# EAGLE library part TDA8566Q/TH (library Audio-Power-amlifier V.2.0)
The TDA8566Q is an integrated class-B output amplifier contained in a 17-lead single-in-line (SIL; bent to DIL) plastic power package. The device contains two amplifiers in a Bridge-Tied Load configuration (BTL). The output power is 2 ´ 25 W in a 4 W load or 2 ´ 40 W in a 2 W load. It has a differential input stage and two diagnostic outputs. The device is primarily developed for car radio applications. The TDA8566TH is an integrated class-B output amplifier contained in a 20-lead small outline plastic package. The device contains 2 amplifiers in a Bridge-Tied Load (BTL) configuration. The output power is 2 ´ 25 W in a 4 W load or 2 ´ 40 W in a 2 W load. It has a differential input stage and 2 diagnostic outputs. The device is primarily developed for car radio applications.
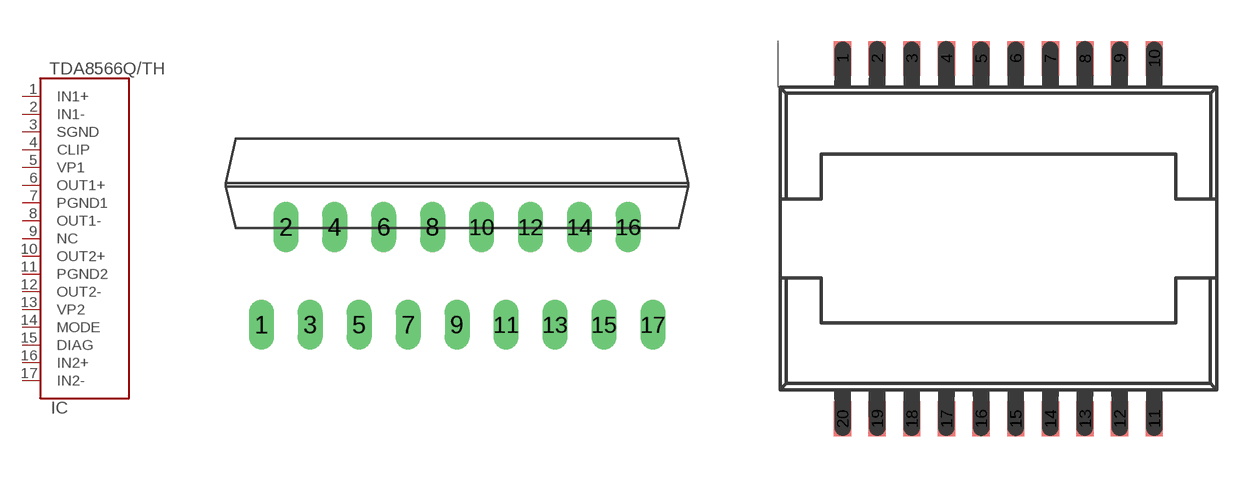
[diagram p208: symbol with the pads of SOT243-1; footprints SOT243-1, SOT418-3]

Designator prefix IC

## TDA8566Q/THTDA8566Q  [SOT243-1]
1  IN1+  in
2  IN1-  in
3  SGND  pwr
4  CLIP
5  VP1  pwr
6  OUT1+  out
7  PGND1  pwr
8  OUT1-  out
9  NC  nc
10  OUT2+  out
11  PGND2  pwr
12  OUT2-  out
13  VP2  pwr
14  MODE  in
15  DIAG  in
16  IN2+  in
17  IN2-  in

## TDA8566Q/THTDA8566TH  [SOT418-3]
1  DIAG  in
2  IN2+  in
3  IN2-  in
6  NC  nc
8  IN1+  in
9  IN1-  in
10  SGND  pwr
11  CLIP
12  VP1  pwr
13  OUT1+  out
14  PGND1  pwr
15  OUT1-  out
16  OUT2+  out
17  PGND2  pwr
18  OUT2-  out
19  VP2  pwr
20  MODE  in

## Footprint SOT243-1 (pad centres in mm)
DBS17P: plastic DIL-bent-SIL power package; 17 leads (lead length 7.7 mm)
drill 0.8 long: 1 -10.16,-5.08; 2 -8.89,0; 3 -7.62,-5.08; 4 -6.35,0; 5 -5.08,-5.08; 6 -3.81,0; 7 -2.54,-5.08; 8 -1.27,0; 9 0,-5.08; 10 1.27,0; 11 2.54,-5.08; 12 3.81,0; 13 5.08,-5.08; 14 6.35,0; 15 7.62,-5.08; 16 8.89,0; 17 10.17,-5.08

## Footprint SOT418-3 (pad centres in mm)
smd 0.635 x 1.27: 1 -5.715,6.615; 2 -4.445,6.615; 3 -3.175,6.615; 4 -1.905,6.615; 5 -0.635,6.615; 6 0.635,6.615; 7 1.905,6.615; 8 3.175,6.615; 9 4.445,6.615; 10 5.715,6.615; 11 5.715,-6.615; 12 4.445,-6.615; 13 3.175,-6.615; 14 1.905,-6.615; 15 0.635,-6.615; 16 -0.635,-6.615; 17 -1.905,-6.615; 18 -3.175,-6.615; 19 -4.445,-6.615; 20 -5.715,-6.615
